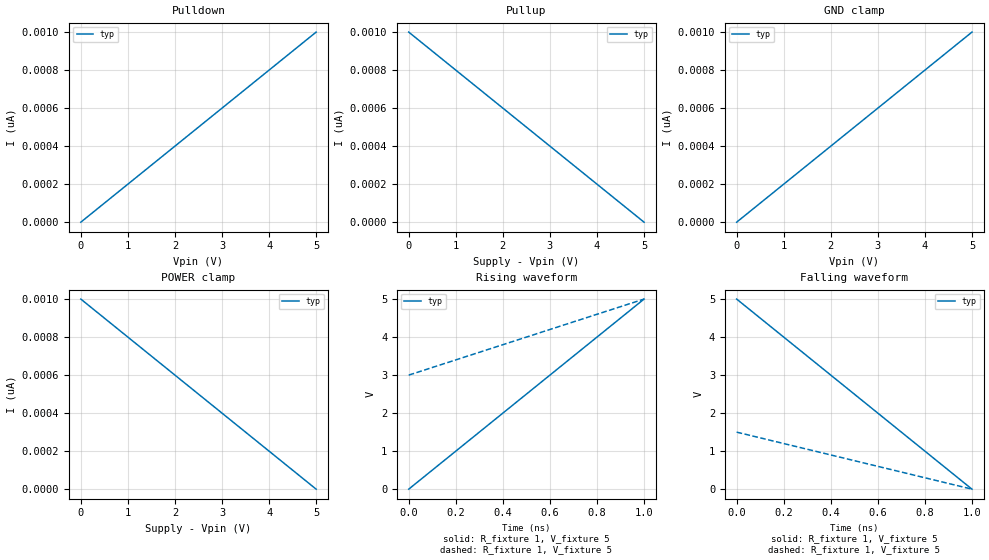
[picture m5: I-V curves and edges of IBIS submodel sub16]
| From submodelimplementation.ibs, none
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| ... Check repetitions and invalid data
[Submodel] sub16
Submodel_type Dynamic_clamp
Submodel_type Bus_hold
[Submodel Spec]
V_trigger_f   1.4   1.2   1.6
V_trigger_r   3.6   2.9   4.3
[Submodel Spec]
V_trigger_f   1.4   1.2   1.6
V_trigger_r   3.6   2.9   4.3
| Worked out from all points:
|   rising waveform, R_fixture 1, V_fixture 5: 20-80 % time 600ps typ, NA min, NA max; typ from 0 V to 5 V
|   rising waveform, R_fixture 1, V_fixture 5: 20-80 % time 600ps typ, NA min, NA max; typ from 3 V to 5 V
|   falling waveform, R_fixture 1, V_fixture 5: 20-80 % time 600ps typ, NA min, NA max; typ from 5 V to 0 V
|   falling waveform, R_fixture 1, V_fixture 5: 20-80 % time 600ps typ, NA min, NA max; typ from 1.5 V to 0 V
[GND Clamp]
0V        0A         NA         NA
5V        1nA        NA         NA
[GND Clamp]
0V        1nA        NA         NA
5V        0A         NA         NA
[POWER Clamp]
0V        1nA        NA         NA
5V        0A         NA         NA
[POWER Clamp]
0V        0A         NA         NA
5V        1nA        NA         NA
[Rising Waveform]
R_fixture = 1
V_fixture = 5
0s        0V         NA         NA
1ns       5V         NA         NA
[Rising Waveform]
R_fixture = 1
V_fixture = 5
0s        3V         NA         NA
1ns       5V         NA         NA
[Falling Waveform]
R_fixture = 1
V_fixture = 5
0s        5V         NA         NA
1ns       0V         NA         NA
[Falling Waveform]
R_fixture = 1
V_fixture = 5
0s        1.5V       NA         NA
1ns       0V         NA         NA
[Ramp]
dV/dt_r		1/1n   NA   NA
dV/dt_f		1/1n   NA   NA
[Ramp]
dV/dt_r		1/1   NA   NA
dV/dt_f		1/1   NA   NA
[Pullup]
0V        1nA        NA         NA
5V        0A         NA         NA
[Pullup]
0V        0A         NA         NA
5V        1nA        NA         NA
[Pulldown]
0V        0A         NA         NA
5V        1nA        NA         NA
[Pulldown]
0V        1nA        NA         NA
5V        0A         NA         NA
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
